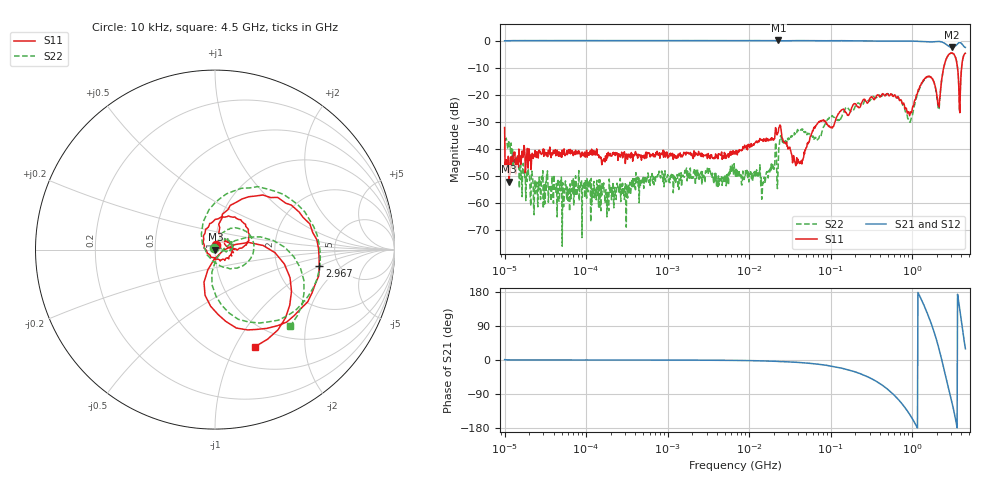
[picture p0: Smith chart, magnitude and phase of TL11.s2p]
!Siglent Technologies,SNA5004A,SNA5XCED5R0097,V1.0.0.2.10.R9
!Date: 2024-11-24 17:26:07
!Data & Calibration Information:
!Freq	S11:F2(ON)	S21:F2(ON)	S12:F2(ON)	S22:F2(ON)
# Hz S DB R 50
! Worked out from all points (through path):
!   1001 points, 10 kHz to 4.5 GHz, reference 50 ohm
!   highest |S21| = 0.11 dB at 22.8 MHz (marker M1); lowest = -2.5 dB at 3.085 GHz (marker M2)
!   group delay of S21, straight-line fit = 427 ps
!   lowest |S11| = -52.3 dB at 11.39 kHz (marker M3), VSWR 1.00, Z = 50.2 - j0.0536 ohm
!   |S11| at or under -10 dB: start of sweep to 2.437 GHz; 3.607 GHz to 4.041 GHz (434.3 MHz wide, 11.4 % of centre)
!   |S22| runs from -76.1 to -4.5 dB; largest |S21 - S12| = 0.022
!   S11 on the Smith chart (normalised r, x): 10 kHz: 1.01, +0.05; 2.967 GHz: 3.55, -1.00; 4.5 GHz: 0.74, -1.21
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10000  -32.16 82.7  -0.01 0.9  -0.02 0.9  -40.04 117.7
11390.22  -52.26 -12.7  0.02 0.3  -0.04 0.2  -39.49 102.9
23920.22  -41.39 3.1  0.06 0.1  0.00 -0.0  -56.63 119.1
87919.76  -42.66 8.2  0.06 0.0  0.00 -0.1  -51.65 -46.7
772988.4  -42.45 16.7  0.06 -0.1  0.01 -0.3  -49.81 -48.2
6708204  -42.03 60.7  0.04 -1.1  -0.03 -1.3  -48.04 -135.1
1.484063e7  -37.29 95.7  0.05 -2.4  -0.02 -2.5  -52.45 -26.4
2.280385e7  -33.76 116.4  0.11 -3.8  0.03 -3.8  -44.75 100.8
3.939519e7  -43.81 138.8  0.06 -6.2  -0.04 -6.4  -32.89 83.8
5.897837e7  -34.12 53.3  0.01 -9.4  -0.05 -9.5  -35.22 99.3
2.313556e8  -24.44 46.5  -0.05 -36.2  -0.12 -36.0  -23.56 58.4
5.185364e8  -20.41 1.1  -0.13 -80.1  -0.19 -79.8  -19.87 16.4
9.314806e8  -27.79 -136.5  -0.13 -143.5  -0.17 -143.1  -30.07 26.6
1.132327e9  -19.92 129.6  -0.18 -174.8  -0.23 -174.4  -21.06 66.6
1.739915e9  -13.76 22.3  -0.42 92.2  -0.48 92.7  -13.78 -14.0
2.087723e9  -23.70 18.3  -0.25 37.1  -0.31 37.6  -25.45 -122.0
2.286891e9  -14.98 77.4  -0.41 4.0  -0.47 4.5  -15.48 113.1
2.966946e9  -4.61 -9.1  -2.43 -97.9  -2.45 -97.0  -4.63 -1.7
3.085101e9  -4.55 -23.9  -2.50 -113.2  -2.53 -112.2  -4.56 -16.4
3.653937e9  -11.68 -102.2  -0.99 165.7  -1.04 166.6  -11.74 -88.8
4.002521e9  -11.40 4.9  -0.93 103.2  -0.97 104.6  -11.62 15.7
4.5e9  -4.66 -67.5  -2.47 29.8  -2.54 31.1  -4.46 -45.3
